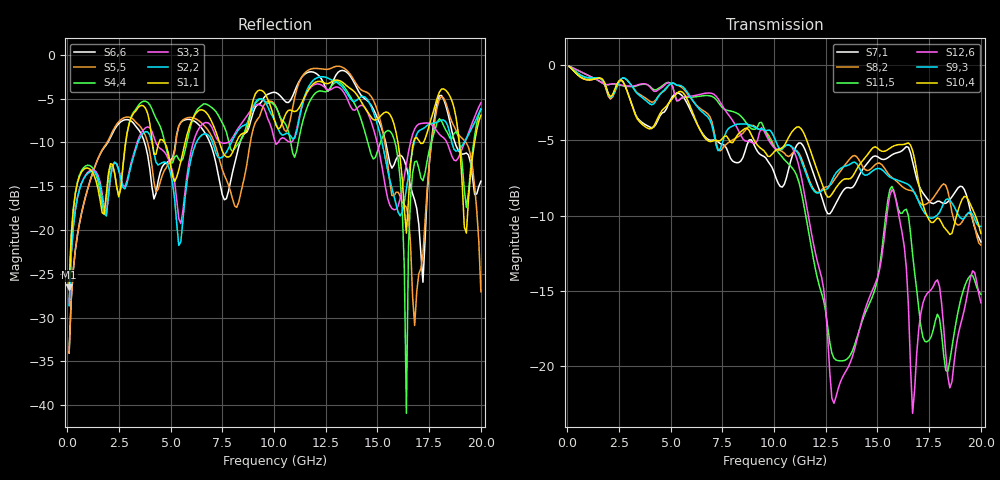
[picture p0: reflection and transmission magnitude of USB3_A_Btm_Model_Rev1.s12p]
! Touchstone file from project USB_Dual_A
! Exported from HFSS 11.1.3
# GHZ S RI R 45.000000
! Terminal data exported
! Port[1] = SSTX_p_MB
! Port[2] = SSTX_n_MB
! Port[3] = SSRX_p_MB
! Port[4] = SSRX_n_MB
! Port[5] = USB2_p_MB
! Port[6] = USB2_n_MB
! Port[7] = SSTX_p_Cable
! Port[8] = SSTX_n_Cable
! Port[9] = SSRX_p_Cable
! Port[10] = SSRX_n_Cable
! Port[11] = USB2_p_Cable
! Port[12] = USB2_n_Cable
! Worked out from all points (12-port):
!   200 points, 100 MHz to 20 GHz, reference 45 ohm
!   strongest paths, dB at 100 MHz, 5.1 GHz, 10.1 GHz, 15.1 GHz, 20 GHz:
!     S10,4: -0.1, -2.2, -5.6, -5.6, -11.2
!     S9,3: -0.1, -1.2, -5.1, -6.9, -10.7
!     S12,6: 0.0, -1.4, -5.6, -13.6, -15.8
!     S11,5: 0.0, -1.4, -5.6, -13.5, -15.3
!     S8,2: -0.1, -1.2, -5.6, -6.5, -12.0
!     S7,1: -0.1, -2.1, -7.5, -6.2, -11.8
!   lowest |S11| = -26.5 dB at 100 MHz (marker M1), VSWR 1.10, Z = 45.9 + j4.2 ohm
!   |S11| at or under -10 dB: start of sweep to 2.836 GHz; 4.705 GHz to 5.706 GHz (1 GHz wide, 19.2 % of centre); 7.362 GHz to 8.182 GHz (819.5 MHz wide, 10.5 % of centre)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
